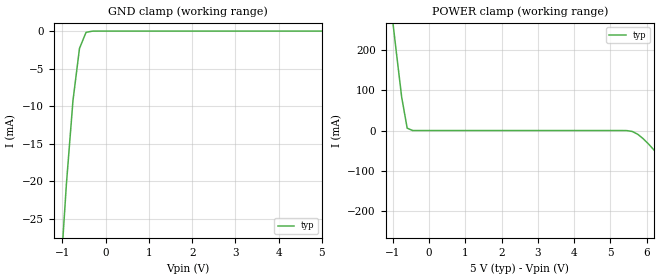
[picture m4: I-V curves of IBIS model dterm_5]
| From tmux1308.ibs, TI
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| dterm_5
[Model]   dterm_5
Model_type   Terminator
|   typ   min   max
C_comp   1.008417e-11   NA   NA
[Voltage Range]   5   NA   NA
[Temperature Range]   27   NA   NA
[Power Clamp Reference]   5   NA   NA
[GND Clamp Reference]   0   NA   NA
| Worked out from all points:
|   GND clamp passes 1 mA (typ) near -0.51 V on its own axis
|   POWER clamp passes 1 mA (typ) near -0.48 V on its own axis
[GND Clamp]
|   Voltage   I(typ)   I(min)   I(max)
-10V      -75.72kA   NA         NA
-1.061V   -33.87mA   NA         NA
-909.1mV  -20.36mA   NA         NA
-757.6mV  -9.269mA   NA         NA
-606.1mV  -2.298mA   NA         NA
-454.5mV  -164.5uA   NA         NA
-303mV    -3.412uA   NA         NA
5V        2.454nA    NA         NA
[POWER Clamp]
|   Voltage   I(typ)   I(min)   I(max)
-5V       1.687A     NA         NA
-1.061V   314.6mA    NA         NA
-909.1mV  197mA      NA         NA
-757.6mV  82.38mA    NA         NA
-606.1mV  5.837mA    NA         NA
-454.6mV  8.723uA    NA         NA
5.606V    -2.298mA   NA         NA
5.909V    -20.36mA   NA         NA
6.364V    -64.93mA   NA         NA
7.879V    -249mA     NA         NA
8.03V     -487.9mA   NA         NA
10V       -20.06kA   NA         NA
